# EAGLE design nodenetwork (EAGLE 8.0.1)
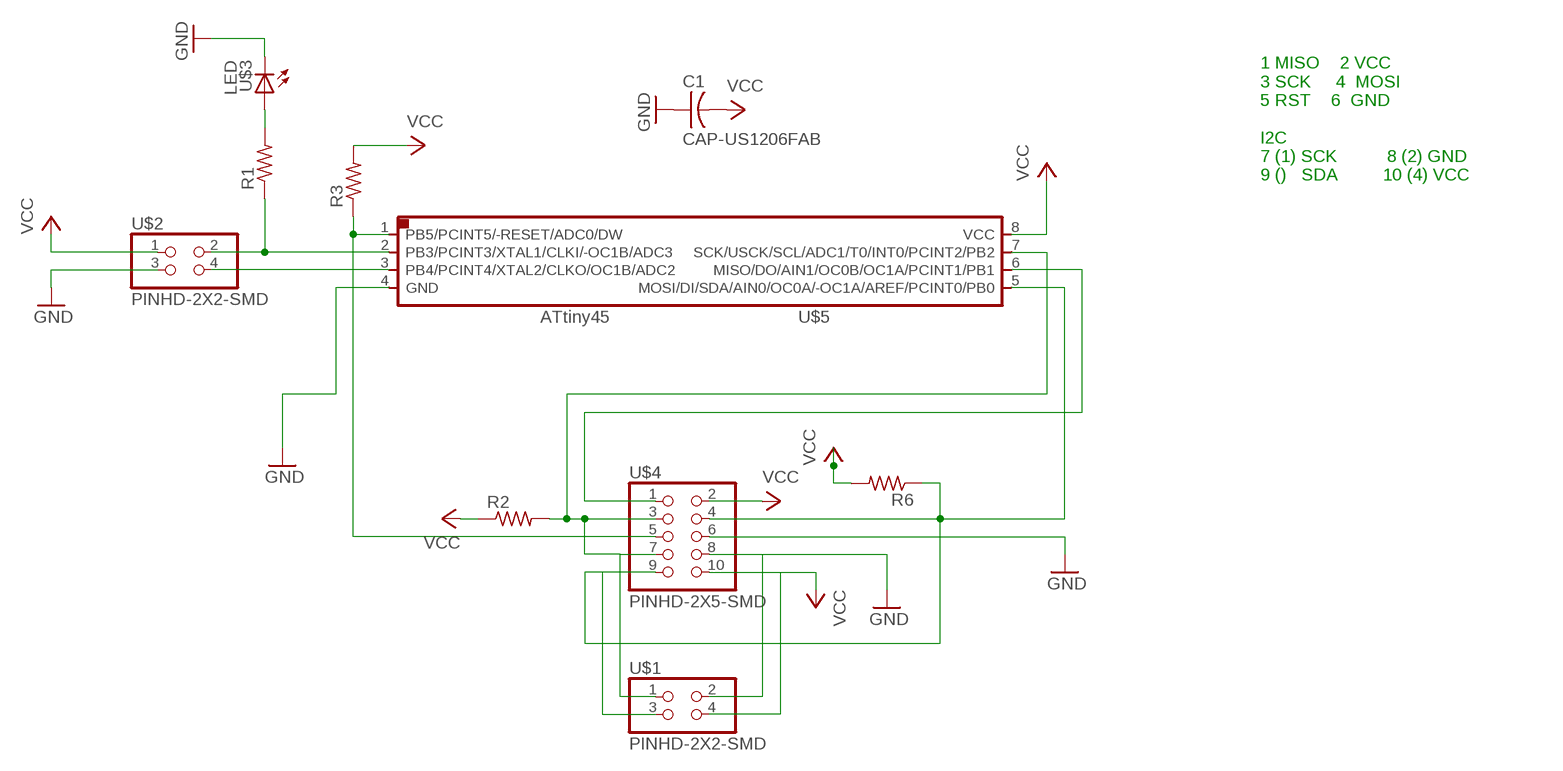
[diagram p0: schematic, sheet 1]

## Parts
C1  CAP-US1206FAB  [C1206FAB]
R1  RES-US1206FAB  [R1206FAB]
R2  RES-US1206FAB  [R1206FAB]
R3  RES-US1206FAB  [R1206FAB]
R6  RES-US1206FAB  [R1206FAB]
U$1  PINHD-2X2-SMD  [2X02SMD]
U$2  PINHD-2X2-SMD  [2X02SMD]
U$3  LED  [LED1206]
U$4  PINHD-2X5-SMD  [2X05SMD]
U$5  ATTINY45SI  [SOIC8]

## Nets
GND: C1.1 U$1.2 U$2.3 U$3.2(C) U$4.6 U$4.8 U$5.4(GND)
N$1: U$2.4 U$5.3(PB4/PCINT4/XTAL2/CLKO/OC1B/ADC2)
N$2: R1.1 U$2.2 U$5.2(PB3/PCINT3/XTAL1/CLKI/-OC1B/ADC3)
N$3: R1.2 U$3.1(A)
N$7: U$4.1 U$5.6(MISO/DO/AIN1/OC0B/OC1A/PCINT1/PB1)
N$8: R6.1 U$1.3 U$4.4 U$4.9 U$5.5(MOSI/DI/SDA/AIN0/OC0A/-OC1A/AREF/PCINT0/PB0)
N$9: R3.1 U$4.5 U$5.1(PB5/PCINT5/-RESET/ADC0/DW)
N$10: R2.2 U$1.1 U$4.3 U$4.7 U$5.7(SCK/USCK/SCL/ADC1/T0/INT0/PCINT2/PB2)
VCC: C1.2 R2.1 R3.2 R6.2 U$1.4 U$2.1 U$4.2 U$4.10 U$5.8(VCC)

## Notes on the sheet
- 1 MISO    2 VCC
  3 SCK     4  MOSI
  5 RST    6  GND
  
  I2C
  7 (1) SCK          8 (2) GND
  9 ()   SDA         10 (4) VCC

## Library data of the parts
C1 = fab:CAP-US
R1-R3 R6 = fab:RES-US: Resistor (US Symbol)
U$1 U$2 = fab:PINHD-2X2-SMD
U$3 = fab:LED: LED
U$4 = fab:PINHD-2X5-SMD
U$5 = fab:ATTINY45

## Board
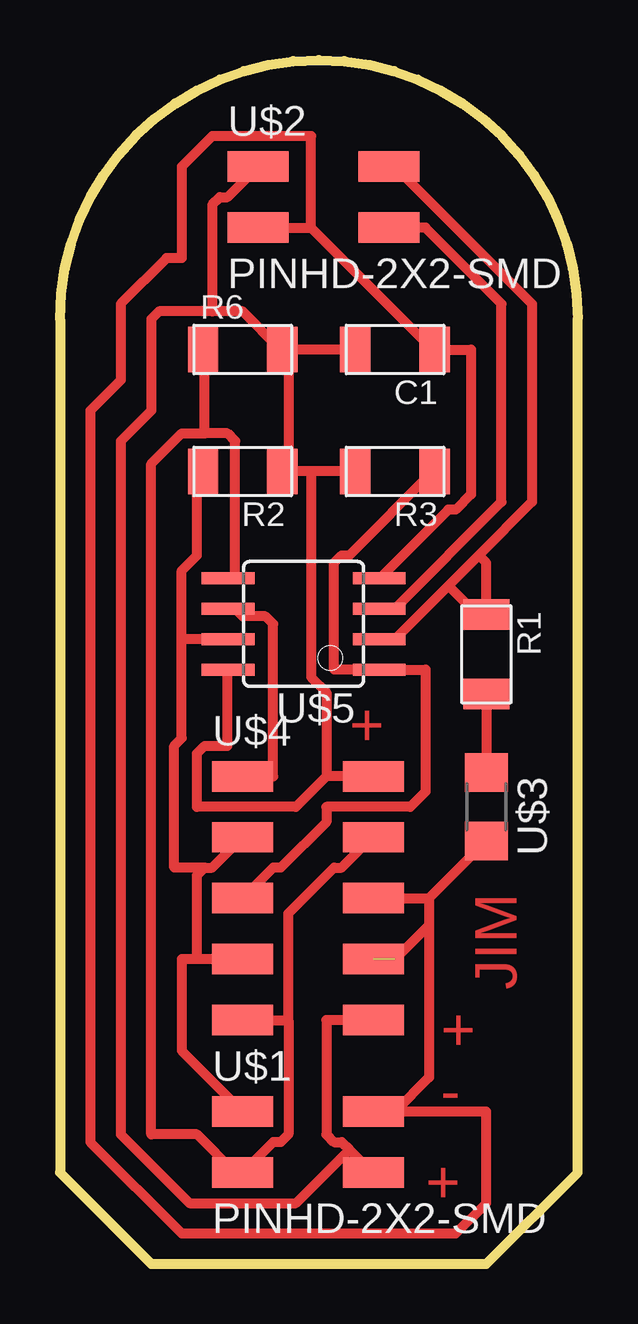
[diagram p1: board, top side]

Size 21.59 x 50.16 mm. Coordinates in mm from the lower left corner, seen from the top.
Outline: 0,39.37 0,3.81 3.81,0 17.78,0 21.59,3.81 21.59,39.37 arc180 0,39.37
Copper layers (1*16): Top 0.035mm / dielectric 1.5mm / Bottom 0.035mm
Design rules "default *": minimum track width 16mil, minimum drill 24mil, track to track 16mil, track to pad 16mil, pad to pad 16mil, via to via 16mil, smd to smd 8mil, copper to edge 40mil, drill to drill 8mil, minimum pad ring 10mil, minimum via ring 8mil, stop-mask expansion 4mil, vias tented up to drill 0mil, thermal gap 10mil

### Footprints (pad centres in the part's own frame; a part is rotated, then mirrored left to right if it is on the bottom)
C1206FAB = smd 1.27 x 1.905: 1 -1.651,0; 2 1.651,0
R1206FAB = smd 1.27 x 1.905: 1 -1.651,0; 2 1.651,0
2X02SMD = smd 2.54 x 1.27: 1 -2.54,1.27; 2 2.92,1.27; 3 -2.54,-1.27; 4 2.92,-1.27
LED1206 = smd 1.6 x 1.803: 1 -1.422,0; 2 1.422,0
2X05SMD = smd 2.54 x 1.27: 1 -2.54,2.54; 2 2.92,2.54; 3 -2.54,0; 4 2.92,0; 5 -2.54,-2.54; 6 2.92,-2.54; 7 -2.54,-5.08; 8 2.92,-5.08; 9 -2.54,-7.62; 10 2.92,-7.62
SOIC8 = smd 0.5 x 2.2: 1 -1.905,-3.154; 2 -0.645,-3.154; 3 0.625,-3.154; 4 1.895,-3.154; 5 1.905,3.154; 6 0.635,3.154; 7 -0.635,3.154; 8 -1.905,3.154

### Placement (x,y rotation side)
C1  13.97,38.1 180 top
R1  17.78,25.4 270 top
R2  7.62,33.02 180 top
R3  13.97,33.02 180 top
R6  7.62,38.1 0 top
U$1  10.16,5.08 0 top
U$2  10.79,44.45 0 top
U$3  17.78,19.05 270 top
U$4  10.16,17.78 0 top
U$5  10.16,26.67 90 top

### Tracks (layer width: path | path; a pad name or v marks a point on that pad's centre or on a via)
GND  (1 unrouted)
  Top 0.406: 10.48,43.18 15.56,38.1 C1.1 17.14,38.1 17.14,32.07 16.51,31.43 16.19,31.43 13.34,28.57 U$5.4 | U$2.3 10.48,43.18 | 10.48,43.18 10.48,46.99 6.35,46.99 5.08,45.72 5.08,41.91 4.45,41.91 2.54,40 2.54,36.83 1.27,35.56 1.27,5.08 5.08,1.27 16.51,1.27 17.78,2.54 17.78,6.35 13.97,6.35 | 13.97,6.35 U$1.2 | U$4.6 15.39,15.24 | 15.39,15.24 U$3.2 | 15.39,15.24 15.39,14.12 | 15.39,14.12 13.97,12.7 | 15.39,14.12 15.39,7.77 13.97,6.35
N$1
  Top 0.406: U$5.3 13.96,27.3 18.41,31.75 18.41,40 15.24,43.18 U$2.4
N$2
  Top 0.406: U$5.2 13.34,26.04 13.97,26.04 16.19,28.26 | U$2.2 13.97,45.72 19.68,40 19.68,31.75 17.46,29.53 | 17.46,29.53 16.19,28.26 | 16.19,28.26 17.4,27.05 R1.1 17.78,29.21 17.46,29.53
N$3
  Top 0.406: R1.2 U$3.1
N$7
  Top 0.406: U$4.1 8.89,20.32 8.89,26.67 8.57,26.99 7.62,26.99 7.3,27.3 U$5.6
N$8
  Top 0.406: 6.03,34.61 6.03,38.1 R6.1 | 6.03,34.61 6.99,34.61 7.3,34.29 7.3,28.57 U$5.5 | 9.53,10.16 9.53,5.4 9.21,5.08 8.89,5.08 U$1.3 7.3,3.81 5.71,5.4 3.81,5.4 3.81,33.34 5.08,34.61 6.03,34.61 | U$4.9 9.53,10.16 | 9.53,10.16 9.53,14.61 11.43,16.51 11.75,16.51 13.02,17.78 U$4.4
N$9
  Top 0.406: R3.1 15.56,33.02 12.07,29.53 11.75,29.53 11.43,29.21 11.43,24.77 U$5.1 15.24,24.77 15.24,19.68 14.61,19.05 11.11,19.05 11.11,18.41 9.21,16.51 8.89,16.51 U$4.5
N$10
  Top 0.406: 5.08,26.04 5.08,28.89 5.71,29.53 5.71,33.02 R2.2 | U$5.7 5.08,26.04 | U$1.1 5.08,8.89 5.08,12.7 5.71,12.7 | U$4.7 5.71,12.7 | U$4.3 6.35,16.51 6.03,16.51 | 6.03,16.51 5.71,16.19 5.71,12.7 | 5.08,26.04 5.08,21.91 4.76,21.59 4.76,16.51 6.03,16.51
VCC
  Top 0.406: 11.11,20.32 9.84,19.05 5.71,19.05 5.71,21.27 6.03,21.59 6.99,21.59 6.99,24.77 U$5.8 | U$4.2 11.11,20.32 | 12.07,4.76 11.75,5.08 11.43,5.08 11.11,5.4 11.11,10.16 U$4.10 | 12.07,4.76 13.02,3.81 U$1.4 | R3.2 10.48,33.02 | 10.48,33.02 9.53,33.02 | C1.2 9.53,38.1 | U$2.1 6.99,44.45 6.67,44.45 6.35,44.13 6.35,39.69 | 6.35,39.69 7.62,39.69 9.21,38.1 R6.2 9.53,38.1 | 9.53,38.1 9.53,33.02 | 9.53,33.02 R2.1 | 12.07,4.76 9.84,2.54 5.4,2.54 2.54,5.4 2.54,34.29 3.81,35.56 3.81,39.37 4.13,39.69 6.35,39.69 | 11.11,20.32 11.11,23.81 10.48,24.45 10.48,33.02

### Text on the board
Top: + | JIM | + | - | +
